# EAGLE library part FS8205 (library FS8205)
DUAL N-CHANNEL ENHANCEMENT MODE POWER MOFSET Source: Datasheet
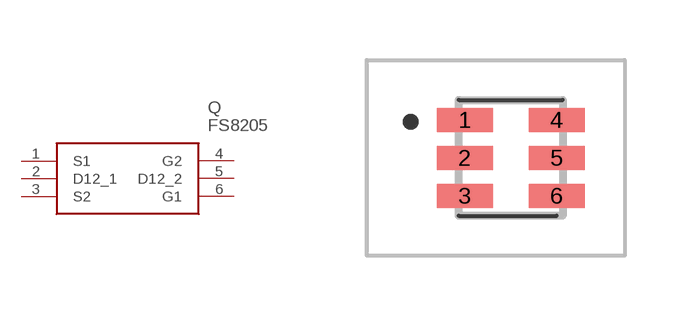
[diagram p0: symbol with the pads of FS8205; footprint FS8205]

Designator prefix Q

## FS8205 (Description: DUAL N-CHANNEL ENHANCEMENT MODE POWER MOFSET; Height: 1mm; Manufacturer_Name: Fortune Semiconductor Corporation; Manufacturer_Part_Number: FS8205)  [FS8205]
1  S1
2  D12_1
3  S2
4  G2
5  D12_2
6  G1

## Footprint FS8205 (pad centres in mm)
FS8205
smd 1.4 x 0.6: 1 -0.5,0.95; 2 -0.5,0; 3 -0.5,-0.95; 4 1.8,0.95; 5 1.8,0; 6 1.8,-0.95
